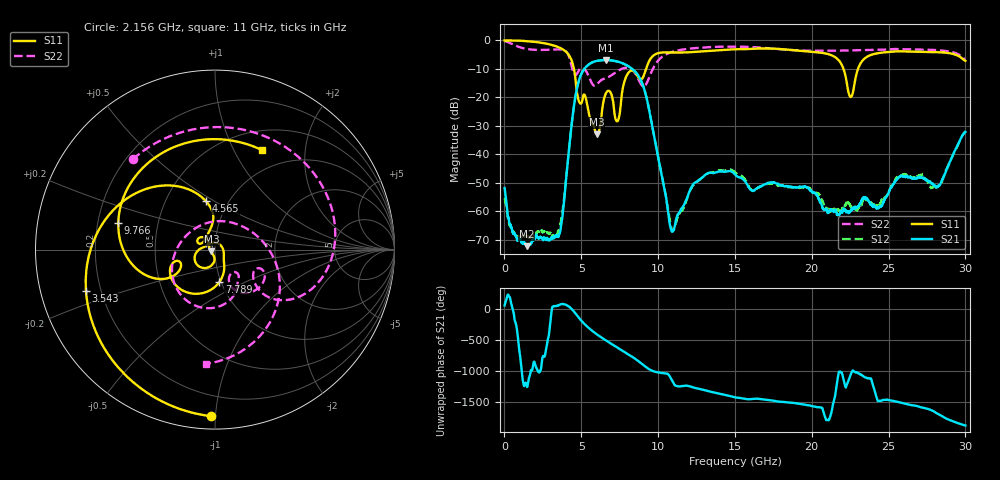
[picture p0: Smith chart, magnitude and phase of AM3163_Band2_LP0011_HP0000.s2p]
!Agilent Technologies,E8364B,MY43040894,A.07.50.67
!Agilent E8364B: A.07.50.67
!Date: Thursday, August 20, 2020 12:04:45
!Correction: S11(Full 2 Port(1,2))
!S21(Full 2 Port(1,2))
!S12(Full 2 Port(1,2))
!S22(Full 2 Port(1,2))
!S2P File: Measurements: S11, S21, S12, S22:
# Hz S  dB  R 50
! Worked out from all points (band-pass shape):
!   3201 points, 10 MHz to 30 GHz, reference 50 ohm
!   highest |S21| = -6.90 dB at 6.608 GHz (marker M1); lowest = -72.3 dB at 1.463 GHz (marker M2)
!   |S21| within 3 dB of the highest: 5.215 GHz to 8.288 GHz (3.074 GHz wide, 45.5 % of centre)
!   lowest |S11| = -33.0 dB at 6.017 GHz (marker M3), VSWR 1.05, Z = 48 - j0.863 ohm
!   |S11| at or under -10 dB: 4.524 GHz to 9.217 GHz (4.693 GHz wide, 68.3 % of centre); 22.07 GHz to 23.01 GHz (945.2 MHz wide, 4.19 % of centre)
!   |S22| runs from -16.2 to -0.3 dB; largest |S21 - S12| = 0.0025
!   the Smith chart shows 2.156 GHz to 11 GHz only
!   S11 on the Smith chart (normalised r, x): 2.156 GHz: 0.07, -0.97; 3.543 GHz: 0.14, -0.15; 4.565 GHz: 0.79, +0.46; 7.789 GHz: 0.98, -0.37; 9.766 GHz: 0.29, +0.12; 11 GHz: 0.73, +1.30
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1e7  -0.02 -2.9  -51.86 63.0  -55.40 129.2  -0.26 -10.9
6.004281e8  -0.05 -24.7  -67.87 -59.8  -67.34 77.6  -1.57 -88.0
1.462641e9  -0.26 -61.0  -72.25 -170.7  -68.66 167.4  -3.00 -175.1
2.156159e9  -0.64 -91.3  -69.15 87.8  -67.22 108.9  -3.34 132.3
3.543197e9  -2.45 -162.4  -68.27 67.5  -66.79 -135.9  -3.16 34.1
4.564731e9  -11.24 100.6  -21.49 -48.2  -21.50 -48.4  -11.88 -33.6
5.014581e9  -21.94 151.6  -11.64 173.8  -11.66 173.6  -9.77 -35.7
6.017372e9  -33.01 -156.3  -7.20 -44.6  -7.21 -44.8  -15.39 -47.8
6.6078e9  -18.52 -119.9  -6.90 -142.9  -6.90 -143.0  -13.24 -54.3
7.348178e9  -28.38 58.3  -7.42 103.6  -7.45 103.4  -10.81 -71.7
7.788656e9  -14.80 -82.3  -8.26 36.6  -8.29 36.6  -9.71 -94.0
9.766122e9  -5.05 164.5  -34.49 73.9  -34.35 73.0  -8.91 -15.5
1.000979e10  -4.47 142.7  -41.28 59.1  -41.05 57.2  -7.04 -36.8
1.100321e10  -4.25 64.6  -66.34 -108.7  -66.56 -99.5  -3.89 -94.5
1.319623e10  -3.72 -66.9  -46.81 123.1  -46.81 127.2  -2.41 -172.8
1.5005e10  -3.13 -143.9  -47.05 18.0  -46.32 19.9  -2.17 127.5
1.768536e10  -2.94 93.9  -50.25 -45.8  -50.64 -47.5  -3.00 28.3
2.000958e10  -4.02 -30.5  -53.21 -123.6  -52.82 -124.3  -3.63 -52.5
2.253999e10  -19.88 -104.6  -59.98 28.8  -58.38 -169.3  -3.51 -123.7
2.500479e10  -4.09 -151.7  -53.44 -26.0  -53.59 -27.7  -3.19 175.9
2.829432e10  -4.18 105.6  -50.97 98.0  -50.88 102.0  -3.48 88.0
3e10  -7.19 43.1  -32.14 -76.6  -31.94 -77.1  -6.77 35.8
